| / 7\'7
| \ \   Xilinx Inc.
| / /
| \_\/.\   IBIS Models for VIRTEX-5
[IBIS ver]   3.2
[File name]   dlpc410.ibs
[File Rev]   1.8
[Date]   December 31, 2012
[Source]   Derived from spice models, rev0.20, dated 08/10/2005 using
   hspice 2005.03
[Notes]   Xilinx IBIS file for VIRTEX-5 I/O standards.
   All models are preliminary.
   The version of IBISCHK used is ibischk4.
   Ibis models were generated using S2IBIS3.
   To accurately model package parasitics, please include in
   your simulation a 50-65 ohm transmission line with 10-200ps of
   delay. For additional information, please see this Answer
   Record: http://support.xilinx.com/techdocs/11754.htm
   NOTE: This file is compliant with IBIS Version 3.2, but it
   may not implement all approved 3.2 features.
   NOTE:  Newer versions of the buffer models may be available.
   Check the web (http://www.xilinx.com/support/sw_ibis.htm) for
   the latest file revision.  However, please be aware that the
   web files are not compatible for use with IBISWriter, and
   must be manually annotated, should their use be preferred.
[Disclaimer] The data in this file is derived from SPICE simulations using
   modeling information extracted from the target process. While
   a great deal of care has been taken to provide information
   that is accurate, this model is considered preliminary as it
   has not been verified by actual silicon measurement. Treat the
   data in this model as preliminary until actual silicon
   verification is performed.
[Copyright]   Copyright 2006, Xilinx Inc., All rights reserved
|   Component VIRTEX-5
[Component]   VIRTEX-5
[Manufacturer]   Xilinx Inc.
[Package]
| For Package Type ff676
| variable   typ   min   max
R_pkg   253.6m   20.7m   604.1m
L_pkg   3.14nH   0.75nH   7.16nH
C_pkg   2.45pF   1.10pF   4.60pF
[Pin]  signal_name   model_name   R_pin   L_pin   C_pin
F7	APPS_CNTL_DPN   NC
E7 	APPS_CNTL_DPP   NC
AC13	ARSTZ   LVCMOS25_S_12_I
M14 	AVDD_0   NC
M13	AVSS_0   NC
E12 	BLKAD_0   LVCMOS25_S_12_I
D13	BLKAD_1   LVCMOS25_S_12_I
E13	BLKAD_2   LVCMOS25_S_12_I
F13	BLKAD_3   LVCMOS25_S_12_I
H13	BLKMD_0   LVCMOS25_S_12_I
H14	BLKMD_1   LVCMOS25_S_12_I
AD13	CLKIN_R   LVCMOS25_S_12_I
G19	COMP_DATA   LVCMOS25_S_12_I
N18	CS_B_0   NC
W11 	D_OUT_BUSY_0   NC
E1	DAD_A_ADDR0   LVCMOS25_F_12_O
E2	DAD_A_ADDR1   LVCMOS25_F_12_O
E3	DAD_A_ADDR2   LVCMOS25_F_12_O
F3 	DAD_A_ADDR3   LVCMOS25_F_12_O
C1	DAD_A_MODE0   LVCMOS25_F_12_O
D1	DAD_A_MODE1   LVCMOS25_F_12_O
AE3	DAD_A_SCPENZ   LVCMOS25_F_12_O
AB12	DAD_A_SEL0   LVCMOS25_F_12_O
AC12 	DAD_A_SEL1   LVCMOS25_F_12_O
AF3 	DAD_A_STROBE   LVCMOS25_F_12_O
E26	DAD_B_ADDR0   LVCMOS25_F_12_O
E25 	DAD_B_ADDR1   LVCMOS25_F_12_O
F25   DAD_B_ADDR2   LVCMOS25_F_12_O
F24	DAD_B_ADDR3   LVCMOS25_F_12_O
D26	DAD_B_MODE0   LVCMOS25_F_12_O
D25	DAD_B_MODE1   LVCMOS25_F_12_O
AB19	DAD_B_SCPENZ   LVCMOS25_F_12_O
R22	DAD_B_SEL0   LVCMOS25_F_12_O
R23	DAD_B_SEL1   LVCMOS25_F_12_O
AB20	DAD_B_STROBE   LVCMOS25_F_12_O
AF4	DAD_INIT   LVCMOS25_F_12_O
AF5	DAD_OEZ   LVCMOS25_F_12_O
L23	DDC_B11_VRN   NC
L22	DDC_B11_VRP   NC
C22	DDC_B11_VRP   NC
M5	DDC_B12_VRN   NC
M6	DDC_B12_VRP   NC
D23	DDC_B15_VRN   NC
A4	DDC_B16_VRN   NC
A5	DDC_B16_VRP   NC
B21	DDC_DCLK_A_DPN   LVDS_25
C21	DDC_DCLK_A_DPP   LVDS_25_I
A7	DDC_DCLK_B_DPN   LVDS_25
B7	DDC_DCLK_B_DPP  	LVDS_25_I
K20	DDC_DCLK_C_DPN   LVDS_25
K21	DDC_DCLK_C_DPP   LVDS_25_I
L5	DDC_DCLK_D_DPN   LVDS_25
K5	DDC_DCLK_D_DPP   LVDS_25_I
N1	DDC_DCLKOUT_A_DPN  	LVDS_25
M1 	DDC_DCLKOUT_A_DPP 	LVDS_25_O
Y5	DDC_DCLKOUT_B_DPN 	LVDS_25
Y6 	DDC_DCLKOUT_B_DPP 	LVDS_25_O
AA22	DDC_DCLKOUT_C_DPN 	LVDS_25
AB22	DDC_DCLKOUT_C_DPP  	LVDS_25_O
M26	DDC_DCLKOUT_D_DPN  	LVDS_25
M25 	DDC_DCLKOUT_D_DPP 	LVDS_25_O
A15	DDC_DIN_A0_DPN  	LVDS_25
A14	DDC_DIN_A0_DPP  	LVDS_25_I
B14 	DDC_DIN_A1_DPN  	LVDS_25
C14	DDC_DIN_A1_DPP  	LVDS_25_I
A22	DDC_DIN_A10_DPN 	LVDS_25
B22	DDC_DIN_A10_DPP   LVDS_25_I
A24	DDC_DIN_A11_DPN 	LVDS_25
A23	DDC_DIN_A11_DPP   LVDS_25_I
C23	DDC_DIN_A12_DPN 	LVDS_25
B24	DDC_DIN_A12_DPP   LVDS_25_I
C24	DDC_DIN_A13_DPN   LVDS_25
D24	DDC_DIN_A13_DPP 	LVDS_25_I
A25	DDC_DIN_A14_DPN 	LVDS_25
B25	DDC_DIN_A14_DPP 	LVDS_25_I
C26	DDC_DIN_A15_DPN 	LVDS_25
B26	DDC_DIN_A15_DPP 	LVDS_25_I
B16	DDC_DIN_A2_DPN  	LVDS_25
B15 	DDC_DIN_A2_DPP   LVDS_25_I
C16	DDC_DIN_A3_DPN  	LVDS_25
D16 	DDC_DIN_A3_DPP   LVDS_25_I
A17	DDC_DIN_A4_DPN  	LVDS_25
B17	DDC_DIN_A4_DPP  	LVDS_25_I
C17	DDC_DIN_A5_DPN  	LVDS_25
D18 	DDC_DIN_A5_DPP   LVDS_25_I
A19	DDC_DIN_A6_DPN  	LVDS_25
A18 	DDC_DIN_A6_DPP   LVDS_25_I
C18	DDC_DIN_A7_DPN   LVDS_25
B19	DDC_DIN_A7_DPP  	LVDS_25_I
D19	DDC_DIN_A8_DPN  	LVDS_25
C19 	DDC_DIN_A8_DPP   LVDS_25_I
B20	DDC_DIN_A9_DPN   LVDS_25
A20	DDC_DIN_A9_DPP   LVDS_25_I
A12	DDC_DIN_B0_DPN   LVDS_25
A13	DDC_DIN_B0_DPP   LVDS_25_I
B12	DDC_DIN_B1_DPN   LVDS_25
C13	DDC_DIN_B1_DPP   LVDS_25_I
B6	DDC_DIN_B10_DPN 	LVDS_25
B5	DDC_DIN_B10_DPP   LVDS_25_I
D4	DDC_DIN_B11_DPN 	LVDS_25
D3	DDC_DIN_B11_DPP  	LVDS_25_I
B4	DDC_DIN_B12_DPN 	LVDS_25
C4	DDC_DIN_B12_DPP 	LVDS_25_I
C3	DDC_DIN_B13_DPN   LVDS_25
C2	DDC_DIN_B13_DPP   LVDS_25_I
A3	DDC_DIN_B14_DPN  	LVDS_25
A2	DDC_DIN_B14_DPP   LVDS_25_I
B2	DDC_DIN_B15_DPN   LVDS_25
B1	DDC_DIN_B15_DPP   LVDS_25_I
D10	DDC_DIN_B2_DPN   LVDS_25
D11	DDC_DIN_B2_DPP   LVDS_25_I
C12	DDC_DIN_B3_DPN   LVDS_25
C11	DDC_DIN_B3_DPP   LVDS_25_I
A10	DDC_DIN_B4_DPN   LVDS_25
B11	DDC_DIN_B4_DPP   LVDS_25_I
D9	DDC_DIN_B5_DPN   LVDS_25
C9	DDC_DIN_B5_DPP   LVDS_25_I
B10	DDC_DIN_B6_DPN   LVDS_25
B9	DDC_DIN_B6_DPP   LVDS_25_I
A8	DDC_DIN_B7_DPN   LVDS_25
A9	DDC_DIN_B7_DPP   LVDS_25_I
D6	DDC_DIN_B8_DPN   LVDS_25
D5	DDC_DIN_B8_DPP   LVDS_25_I
C7	DDC_DIN_B9_DPN   LVDS_25
C6	DDC_DIN_B9_DPP   LVDS_25_I
E20	DDC_DIN_C0_DPN   LVDS_25
E21	DDC_DIN_C0_DPP   LVDS_25_I
F20	DDC_DIN_C1_DPN   LVDS_25
G20	DDC_DIN_C1_DPP  	LVDS_25_I
M19	DDC_DIN_C10_DPN  	LVDS_25
M20	DDC_DIN_C10_DPP  	LVDS_25_I
M21	DDC_DIN_C11_DPN   LVDS_25
M22	DDC_DIN_C11_DPP   LVDS_25_I
N19	DDC_DIN_C12_DPN   LVDS_25
P19	DDC_DIN_C12_DPP   LVDS_25_I
N21	DDC_DIN_C13_DPN   LVDS_25
N22	DDC_DIN_C13_DPP  	LVDS_25_I
P20	DDC_DIN_C14_DPN   LVDS_25
P21	DDC_DIN_C14_DPP  	LVDS_25_I
N23	DDC_DIN_C15_DPN   LVDS_25
P23	DDC_DIN_C15_DPP   LVDS_25_I
H19	DDC_DIN_C2_DPN  	LVDS_25
J19	DDC_DIN_C2_DPP   LVDS_25_I
E23	DDC_DIN_C3_DPN   LVDS_25
E22	DDC_DIN_C3_DPP   LVDS_25_I
F23	DDC_DIN_C4_DPN   LVDS_25
F22	DDC_DIN_C4_DPP   LVDS_25_I
G22	DDC_DIN_C5_DPN   LVDS_25
G21	DDC_DIN_C5_DPP   LVDS_25_I
J20	DDC_DIN_C6_DPN   LVDS_25
J21	DDC_DIN_C6_DPP   LVDS_25_I
H22	DDC_DIN_C7_DPN   LVDS_25
H21	DDC_DIN_C7_DPP   LVDS_25_I
J23	DDC_DIN_C8_DPN   LVDS_25
H23	DDC_DIN_C8_DPP   LVDS_25_I
K22	DDC_DIN_C9_DPN   LVDS_25
K23	DDC_DIN_C9_DPP   LVDS_25_I
T3	DDC_DIN_D0_DPN  	LVDS_25
R3	DDC_DIN_D0_DPP   LVDS_25_I
R5	DDC_DIN_D1_DPN   LVDS_25
R6	DDC_DIN_D1_DPP   LVDS_25_I
H7	DDC_DIN_D10_DPN   LVDS_25
J6	DDC_DIN_D10_DPP 	LVDS_25_I
G4	DDC_DIN_D11_DPN   LVDS_25
H4	DDC_DIN_D11_DPP   LVDS_25_I
G5	DDC_DIN_D12_DPN   LVDS_25
H6	DDC_DIN_D12_DPP 	LVDS_25_I
G7	DDC_DIN_D13_DPN   LVDS_25
G6	DDC_DIN_D13_DPP 	LVDS_25_I
F4	DDC_DIN_D14_DPN  	LVDS_25
F5	DDC_DIN_D14_DPP  	LVDS_25_I
E5	DDC_DIN_D15_DPN   LVDS_25
E6	DDC_DIN_D15_DPP   LVDS_25_I
R7	DDC_DIN_D2_DPN  	LVDS_25
P6	DDC_DIN_D2_DPP   LVDS_25_I
N3	DDC_DIN_D3_DPN   LVDS_25
P3	DDC_DIN_D3_DPP  	LVDS_25_I
P4	DDC_DIN_D4_DPN   LVDS_25
P5	DDC_DIN_D4_DPP   LVDS_25_I
N6	DDC_DIN_D5_DPN   LVDS_25
N7	DDC_DIN_D5_DPP  	LVDS_25_I
N4	DDC_DIN_D6_DPN   LVDS_25
M4	DDC_DIN_D6_DPP  	LVDS_25_I
M7	DDC_DIN_D7_DPN   LVDS_25
L7	DDC_DIN_D7_DPP   LVDS_25_I
K7	DDC_DIN_D8_DPN   LVDS_25
K6	DDC_DIN_D8_DPP   LVDS_25_I
J4	DDC_DIN_D9_DPN   LVDS_25
J5	DDC_DIN_D9_DPP   LVDS_25_I
AE2	DDC_DOUT_A0_DPN 	LVDS_25
AF2	DDC_DOUT_A0_DPP 	LVDS_25_O
AD1	DDC_DOUT_A1_DPN  	LVDS_25
AE1	DDC_DOUT_A1_DPP 	LVDS_25_O
K1	DDC_DOUT_A10_DPN 	LVDS_25
L2	DDC_DOUT_A10_DPP 	LVDS_25_O
K2	DDC_DOUT_A11_DPN 	LVDS_25
K3	DDC_DOUT_A11_DPP 	LVDS_25_O
J3	DDC_DOUT_A12_DPN 	LVDS_25
H3	DDC_DOUT_A12_DPP	LVDS_25_O
H2	DDC_DOUT_A13_DPN	LVDS_25
J1	DDC_DOUT_A13_DPP	LVDS_25_O
H1	DDC_DOUT_A14_DPN	LVDS_25
G1	DDC_DOUT_A14_DPP 	LVDS_25_O
G2	DDC_DOUT_A15_DPN 	LVDS_25
F2	DDC_DOUT_A15_DPP 	LVDS_25_O
AC1	DDC_DOUT_A2_DPN   LVDS_25
AC2	DDC_DOUT_A2_DPP   LVDS_25_O
AB1	DDC_DOUT_A3_DPN   LVDS_25
AB2	DDC_DOUT_A3_DPP   LVDS_25_O
Y2	DDC_DOUT_A4_DPN   LVDS_25
AA2	DDC_DOUT_A4_DPP   LVDS_25_O
W1	DDC_DOUT_A5_DPN   LVDS_25
Y1	DDC_DOUT_A5_DPP   LVDS_25_O
V1	DDC_DOUT_A6_DPN 	LVDS_25
V2	DDC_DOUT_A6_DPP   LVDS_25_O
U1	DDC_DOUT_A7_DPN   LVDS_25
U2	DDC_DOUT_A7_DPP   LVDS_25_O
R2	DDC_DOUT_A8_DPN   LVDS_25
T2	DDC_DOUT_A8_DPP   LVDS_25_O
N2	DDC_DOUT_A9_DPN 	LVDS_25
M2	DDC_DOUT_A9_DPP   LVDS_25_O
AE5	DDC_DOUT_B0_DPN   LVDS_25
AE6	DDC_DOUT_B0_DPP   LVDS_25_O
AD3	DDC_DOUT_B1_DPN   LVDS_25
AD4	DDC_DOUT_B1_DPP   LVDS_25_O
W6	DDC_DOUT_B10_DPN  	LVDS_25
W5	DDC_DOUT_B10_DPP 	LVDS_25_O
V7	DDC_DOUT_B11_DPN 	LVDS_25
V6	DDC_DOUT_B11_DPP	LVDS_25_O
U4	DDC_DOUT_B12_DPN 	LVDS_25
V3	DDC_DOUT_B12_DPP	LVDS_25_O
T4	DDC_DOUT_B13_DPN 	LVDS_25
T5	DDC_DOUT_B13_DPP 	LVDS_25_O
U6	DDC_DOUT_B14_DPN 	LVDS_25
U5	DDC_DOUT_B14_DPP	LVDS_25_O
U7	DDC_DOUT_B15_DPN	LVDS_25
T7	DDC_DOUT_B15_DPP 	LVDS_25_O
AD5	DDC_DOUT_B2_DPN 	LVDS_25
AD6   DDC_DOUT_B2_DPP   LVDS_25_O
AC3	DDC_DOUT_B3_DPN 	LVDS_25
AC4	DDC_DOUT_B3_DPP 	LVDS_25_O
AB5	DDC_DOUT_B4_DPN 	LVDS_25
AB6	DDC_DOUT_B4_DPP   LVDS_25_O
AB7	DDC_DOUT_B5_DPN   LVDS_25
AC6	DDC_DOUT_B5_DPP   LVDS_25_O
AA5	DDC_DOUT_B6_DPN   LVDS_25
AA4	DDC_DOUT_B6_DPP   LVDS_25_O
AA7	DDC_DOUT_B7_DPN   LVDS_25
Y7	DDC_DOUT_B7_DPP   LVDS_25_O
Y3	DDC_DOUT_B8_DPN   LVDS_25
W3	DDC_DOUT_B8_DPP   LVDS_25_O
W4	DDC_DOUT_B9_DPN 	LVDS_25
V4	DDC_DOUT_B9_DPP 	LVDS_25_O
T22	DDC_DOUT_C0_DPN   LVDS_25
T23	DDC_DOUT_C0_DPP   LVDS_25_O
R20	DDC_DOUT_C1_DPN   LVDS_25
R21	DDC_DOUT_C1_DPP   LVDS_25_O
Y20	DDC_DOUT_C10_DPN	LVDS_25
Y21	DDC_DOUT_C10_DPP	LVDS_25_O
AA24	DDC_DOUT_C11_DPN	LVDS_25
AA23	DDC_DOUT_C11_DPP	LVDS_25_O
AA19	DDC_DOUT_C12_DPN	LVDS_25
AA20	DDC_DOUT_C12_DPP	LVDS_25_O
AC24	DDC_DOUT_C13_DPN	LVDS_25
AB24	DDC_DOUT_C13_DPP  	LVDS_25_O
AC19	DDC_DOUT_C14_DPN	LVDS_25
AD19	DDC_DOUT_C14_DPP	LVDS_25_O
AC22	DDC_DOUT_C15_DPN	LVDS_25
AC23	DDC_DOUT_C15_DPP	LVDS_25_O
T19	DDC_DOUT_C2_DPN   LVDS_25
T20	DDC_DOUT_C2_DPP   LVDS_25_O
U21	DDC_DOUT_C3_DPN 	LVDS_25
U22	DDC_DOUT_C3_DPP   LVDS_25_O
U20	DDC_DOUT_C4_DPN   LVDS_25
U19	DDC_DOUT_C4_DPP   LVDS_25_O
V23	DDC_DOUT_C5_DPN   LVDS_25
V24	DDC_DOUT_C5_DPP 	LVDS_25_O
V22	DDC_DOUT_C6_DPN 	LVDS_25
V21	DDC_DOUT_C6_DPP   LVDS_25_O
W19	DDC_DOUT_C7_DPN   LVDS_25
V19	DDC_DOUT_C7_DPP 	LVDS_25_O
W23	DDC_DOUT_C8_DPN   LVDS_25
W24	DDC_DOUT_C8_DPP   LVDS_25_O
Y22	DDC_DOUT_C9_DPN 	LVDS_25
Y23	DDC_DOUT_C9_DPP   LVDS_25_O
AB26	DDC_DOUT_D0_DPN   LVDS_25
AC26	DDC_DOUT_D0_DPP   LVDS_25_O
AA25	DDC_DOUT_D1_DPN 	LVDS_25
AB25	DDC_DOUT_D1_DPP   LVDS_25_O
L25	DDC_DOUT_D10_DPN 	LVDS_25
L24	DDC_DOUT_D10_DPP	LVDS_25_O
K26	DDC_DOUT_D11_DPN 	LVDS_25
K25	DDC_DOUT_D11_DPP	LVDS_25_O
J26	DDC_DOUT_D12_DPN 	LVDS_25
J25	DDC_DOUT_D12_DPP  	LVDS_25_O
J24	DDC_DOUT_D13_DPN   LVDS_25
H24	DDC_DOUT_D13_DPP	LVDS_25_O
H26	DDC_DOUT_D14_DPN	LVDS_25
G26	DDC_DOUT_D14_DPP	LVDS_25_O
G25	DDC_DOUT_D15_DPN	LVDS_25
G24	DDC_DOUT_D15_DPP 	LVDS_25_O
Y26	DDC_DOUT_D2_DPN   LVDS_25
Y25	DDC_DOUT_D2_DPP 	LVDS_25_O
W26	DDC_DOUT_D3_DPN   LVDS_25
W25	DDC_DOUT_D3_DPP   LVDS_25_O
U26	DDC_DOUT_D4_DPN   LVDS_25
V26	DDC_DOUT_D4_DPP   LVDS_25_O
U25	DDC_DOUT_D5_DPN  	LVDS_25
U24	DDC_DOUT_D5_DPP   LVDS_25_O
T25	DDC_DOUT_D6_DPN 	LVDS_25
T24	DDC_DOUT_D6_DPP  	LVDS_25_O
R26	DDC_DOUT_D7_DPN   LVDS_25
R25	DDC_DOUT_D7_DPP  	LVDS_25_O
P24	DDC_DOUT_D8_DPN  	LVDS_25
P25	DDC_DOUT_D8_DPP   LVDS_25_O
N24	DDC_DOUT_D9_DPN   LVDS_25
M24	DDC_DOUT_D9_DPP   LVDS_25_O
W18	DDC_M0   NC
Y17	DDC_M1   NC
V18	DDC_M2   NC
R1	DDC_SCTRL_AN   LVDS_25
P1	DDC_SCTRL_AP   LVDS_25_O
AA3	DDC_SCTRL_BN   LVDS_25
AB4	DDC_SCTRL_BP   LVDS_25_O
W20	DDC_SCTRL_CN   LVDS_25
W21	DDC_SCTRL_CP   LVDS_25_O
N26	DDC_SCTRL_DN   LVDS_25
P26	DDC_SCTRL_DP   LVDS_25_O
AB21	DDC_SPARE_0   LVCMOS25_F_12_O
AC21	DDC_SPARE_1   LVCMOS25_F_12_O
F18	DDC_VERSION_0   LVCMOS25_F_12_O
G17	DDC_VERSION_1   LVCMOS25_F_12_O
H18	DDC_VERSION_2   LVCMOS25_F_12_O
AD14	DMD_A_RESET   LVCMOS25_F_12_O
AB14	DMD_A_SCPENZ   LVCMOS25_F_12_O
AA12	DMD_B_RESET   LVCMOS25_S_12
AC14	DMD_B_SCPENZ   NC
AA17	DMD_TYPE_0   LVCMOS25_F_12_O
AC16	DMD_TYPE_1   LVCMOS25_F_12_O
AB17	DMD_TYPE_2   LVCMOS25_F_12_O
AD15	DMD_TYPE_3   LVCMOS25_F_12_O
K10	DONE_DDC   NC
D20	DVALID_A_DPN   LVDS_25
D21	DVALID_A_DPP   LVDS_25_I
C8	DVALID_B_DPN   LVDS_25
D8	DVALID_B_DPP   LVDS_25_I
L19	DVALID_C_DPN   LVDS_25
L20	DVALID_C_DPP   LVDS_25_I
L3	DVALID_D_DPN   LVDS_25
L4	DVALID_D_DPP   LVDS_25_I
R13	DXN_0   NC
R14	DXP_0   NC
Y18	ECP2_FINISHED   LVCMOS25_F_12_O
AD11	ECP2_M_TP0   NC
AD10	ECP2_M_TP1   NC
AB10 	ECP2_M_TP10   LVCMOS25_F_12_O
AA10 	ECP2_M_TP11   LVCMOS25_F_12_O
Y10	ECP2_M_TP12   LVCMOS25_F_12_O
AC11 	ECP2_M_TP13   LVCMOS25_F_12_O
Y12	ECP2_M_TP14   LVCMOS25_F_12_O
Y11	ECP2_M_TP15   LVCMOS25_F_12_O
AB11	ECP2_M_TP16   LVCMOS25_F_12_O
H8 	ECP2_M_TP17   LVCMOS25_F_12_O
H9	ECP2_M_TP18   LVCMOS25_F_12_O
F12	ECP2_M_TP19   LVCMOS25_F_12_O
AD8	ECP2_M_TP2   NC
G11	ECP2_M_TP20   LVCMOS25_F_12_O
G12	ECP2_M_TP21   LVCMOS25_F_12_O
E11  	ECP2_M_TP22   LVCMOS25_F_12_O
E10	ECP2_M_TP23   LVCMOS25_F_12_O
E8 	ECP2_M_TP24   LVCMOS25_F_12_O
F10	ECP2_M_TP25   LVCMOS25_F_12_O
F9 	ECP2_M_TP26   LVCMOS25_F_12_O
F8	ECP2_M_TP27   LVCMOS25_F_12_O
G10	ECP2_M_TP28   LVCMOS25_F_12_O
G9	ECP2_M_TP29   LVCMOS25_F_12_O
AC8	ECP2_M_TP3   LVCMOS25_F_12_O
H11	ECP2_M_TP30   LVCMOS25_F_12_O
H12 	ECP2_M_TP31   LVCMOS25_F_12_O
AC7	ECP2_M_TP4   LVCMOS25_F_12_O
AC9	ECP2_M_TP5   LVCMOS25_F_12_O
AB9	ECP2_M_TP6   LVCMOS25_F_12_O
AA8	ECP2_M_TP7   LVCMOS25_F_12_O
AA9	ECP2_M_TP8   LVCMOS25_F_12_O
Y8  	ECP2_M_TP9   LVCMOS25_F_12_O
A1   GND   GND
A11   GND   GND
A16   GND   GND
A21   GND   GND
A26   GND   GND
A6   GND   GND
AA1   GND   GND
AA11   GND   GND
AA21   GND   GND
AA26   GND   GND
AB18   GND   GND
AB8   GND   GND
AC15   GND   GND
AC25   GND   GND
AC5   GND   GND
AD12   GND   GND
AD2   GND   GND
AD22   GND   GND
AE14   GND   GND
AE19   GND   GND
AE4   GND   GND
AE9   GND   GND
AF1   GND   GND
AF11   GND   GND
AF16   GND   GND
AF21   GND   GND
AF26   GND   GND
AF6   GND   GND
B13   GND   GND
B18   GND   GND
B3   GND   GND
B8   GND   GND
C15   GND   GND
C25   GND   GND
C5   GND   GND
D12   GND   GND
D2   GND   GND
D22   GND   GND
E19   GND   GND
E9   GND   GND
F1   GND   GND
F16   GND   GND
F26   GND   GND
F6   GND   GND
G13   GND   GND
G18   GND   GND
G23   GND   GND
G3   GND   GND
H10   GND   GND
H20   GND   GND
J13   GND   GND
J15   GND   GND
J17   GND   GND
J7   GND   GND
J9   GND   GND
K12   GND   GND
K14   GND   GND
K16   GND   GND
K19   GND   GND
K24   GND   GND
K4   GND   GND
K8   GND   GND
L1   GND   GND
L11   GND   GND
L13   GND   GND
L15   GND   GND
L17   GND   GND
L21   GND   GND
L26   GND   GND
L9   GND   GND
M10   GND   GND
M12   GND   GND
M16   GND   GND
M18   GND   GND
M3   GND   GND
M8   GND   GND
N11   GND   GND
N15   GND   GND
N17   GND   GND
N25   GND   GND
N5   GND   GND
N9   GND   GND
P10   GND   GND
P12   GND   GND
P16   GND   GND
P2   GND   GND
P22   GND   GND
P7   GND   GND
P8   GND   GND
R11   GND   GND
R15   GND   GND
R17   GND   GND
R19   GND   GND
R9   GND   GND
T1   GND   GND
T10   GND   GND
T12   GND   GND
T14   GND   GND
T16   GND   GND
T26   GND   GND
T6   GND   GND
T8   GND   GND
U13   GND   GND
U15   GND   GND
U17   GND   GND
U18   GND   GND
U23   GND   GND
U3   GND   GND
U9   GND   GND
V10   GND   GND
V14   GND   GND
V16   GND   GND
V20   GND   GND
V8   GND   GND
W13   GND   GND
W15   GND   GND
W17   GND   GND
W7   GND   GND
W9   GND   GND
Y14   GND   GND
Y16   GND   GND
Y19   GND   GND
Y24   GND   GND
Y4   GND   GND
L18  	HSWAPEN   NC
AA18   INIT_ACTIVE   LVCMOS25_F_12_O
J11	INTB_DDC   NC
F19	NS_FLIP   LVCMOS25_S_12_I
J18	PROGB_DDC   NC
J10   PROM_CCK_DDC   LVCMOS25_S_12
K11 	PROM_D0_DDC   NC
AC17   PWR_FLOAT   LVCMOS25_S_12_I
P18	RDWR_B   NC
D14   ROWAD_0   LVCMOS25_S_12_I
D15   ROWAD_1   LVCMOS25_S_12_I
G16 	ROWAD_10   LVCMOS25_S_12_I
E15  	ROWAD_2   LVCMOS25_S_12_I
F14   ROWAD_3   LVCMOS25_S_12_I
G14   ROWAD_4   LVCMOS25_S_12_I
E16   ROWAD_5   LVCMOS25_S_12_I
F15   ROWAD_6   LVCMOS25_S_12_I
G15	ROWAD_7   LVCMOS25_S_12_I
E17	ROWAD_8   LVCMOS25_S_12_I
F17   ROWAD_9   LVCMOS25_S_12_I
H17   ROWMD_0   LVCMOS25_S_12_I
H16   ROWMD_1   LVCMOS25_S_12_I
AB16   RST_ACTIVE   LVCMOS25_F_12_O
E18 	RST2BLKZ   LVCMOS25_S_12_I
R18	RSVD_0   NC
T18 	RSVD_0   NC
AB15   SCPCLK   LVCMOS25_F_12_O
AA15   SCPDI   LVCMOS25_S_12_I
AA14   SCPDO   LVCMOS25_F_12_O
Y13   STEPVCC   LVCMOS25_S_12_I
U11   TCK_JTAG   NC
W10   TDO_DDC   NC
V11 	TDO_XCF16DDC   NC
V12	TMS_JTAG   NC
K18 	VBATT_0   NC
J8   VCCAUX   POWER
K17   VCCAUX   POWER
L8   VCCAUX   POWER
M17   VCCAUX   POWER
N8   VCCAUX   POWER
P17   VCCAUX   POWER
R8   VCCAUX   POWER
T17   VCCAUX   POWER
U8   VCCAUX   POWER
V17   VCCAUX   POWER
W16   VCCAUX   POWER
W8   VCCAUX   POWER
H15   VCCINT   POWER
J12   VCCINT   POWER
J14   VCCINT   POWER
J16   VCCINT   POWER
K13   VCCINT   POWER
K15   VCCINT   POWER
K9   VCCINT   POWER
L10   VCCINT   POWER
L12   VCCINT   POWER
L14   VCCINT   POWER
L16   VCCINT   POWER
M11   VCCINT   POWER
M15   VCCINT   POWER
M9   VCCINT   POWER
N10   VCCINT   POWER
N12   VCCINT   POWER
N16   VCCINT   POWER
P11   VCCINT   POWER
P15   VCCINT   POWER
P9   VCCINT   POWER
R10   VCCINT   POWER
R12   VCCINT   POWER
R16   VCCINT   POWER
T11   VCCINT   POWER
T13   VCCINT   POWER
T15   VCCINT   POWER
T9   VCCINT   POWER
U10   VCCINT   POWER
U12   VCCINT   POWER
U14   VCCINT   POWER
U16   VCCINT   POWER
V13   VCCINT   POWER
V15   VCCINT   POWER
V9   VCCINT   POWER
W14   VCCINT   POWER
Y15   VCCINT   POWER
W12   VCCO_0   POWER
Y9   VCCO_0   POWER
C10   VCCO_1   POWER
F11   VCCO_1   POWER
F21   VCCO_11   POWER
H25   VCCO_11   POWER
J22   VCCO_11   POWER
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[Diff Pin]   inv_pin   vdiff   tdelay_typ   tdelay_min   tdelay_max
[Package Model] ff676_xc5vlx30
[Define Package Model]   ff676_xc5vlx30
[Manufacturer]   Xilinx Inc.
[OEM]   Xilinx_K1
[Description]   676 ball organic flipchip
[Number Of Pins]   444
[Pin Numbers]
P20   | 1   P20   D1.245   IO_L19N_SM9N_11
AC17   | 2   AC17  D1.164   IO_L2P_GC_D11_4
F18   | 3   F18   D1.145   IO_L9P_GC_3
B12   | 4   B12   D1.534   IO_L2N_16
T19   | 5   T19   D1.603   IO_L2N_17
H1   | 6   H1   D1.399   IO_L2N_14
B16   | 7   B16   D1.468   IO_L2N_15
G7   | 8   G7   D1.264   IO_L2N_12
E23   | 9   E23   D1.198   IO_L2N_11
K25   | 10   K25   D1.342   IO_L7P_SM2P_13
U6   | 11   U6   D1.671   IO_L3N_18
U21   | 12   U21   D1.605   IO_L3N_17
A12   | 13   A12   D1.536   IO_L3N_16
C16   | 14   C16   D1.470   IO_L3N_15
G2   | 15   G2   D1.401   IO_L3N_14
F4   | 16   F4   D1.266   IO_L3N_12
F23   | 17   F23   D1.200   IO_L3N_11
F10   | 18   F10   D1.140   IO_L6N_GC_3
J18   | 19   J18   D1.26   PROGRAM_B_0
E8   | 20   E8   D1.144   IO_L8N_GC_3
AC4   | 21   AC4   D1.702   IO_L12P_VRN_18
R25   | 22   R25   D1.365   IO_L12P_VRN_13
M5   | 23   M5   D1.297   IO_L12P_VRN_12
L23   | 24   L23   D1.230   IO_L12P_VRN_11
V21   | 25   V21   D1.635   IO_L12P_VRN_17
A4   | 26   A4   D1.567   IO_L12P_VRN_16
D23   | 27   D23   D1.500   IO_L12P_VRN_15
U2   | 28   U2   D1.432   IO_L12P_VRN_14
K22   | 29   K22   D1.227   IO_L10N_CC_SM15N_11
U7   | 30   U7   D1.669   IO_L2N_18
W12   | 31   W12   D1.35   VCCO_0
C10   | 32   C10   C3.1   VCCO_1
AA16   | 33   AA16  C15.2   VCCO_2
D17   | 34   D17   C4.1   VCCO_3
AB13   | 35   AB13  C16.2   VCCO_4
W11   | 36   W11   D1.59   D_OUT_BUSY_0
M21   | 37   M21   D1.233   IO_L13N_11
T25   | 38   T25   D1.368   IO_L13N_13
N6   | 39   N6   D1.300   IO_L13N_12
A22   | 40   A22   D1.503   IO_L13N_15
V1   | 41   V1   D1.435   IO_L13N_14
W20   | 42   W20   D1.638   IO_L13N_17
B6   | 43   B6   D1.570   IO_L13N_16
L25   | 44   L25   D1.341   IO_L6N_SM3N_13
F19   | 45   F19   D1.142   IO_L7N_GC_3
Y18   | 46   Y18   D1.97   IO_L1N_CC_A24_2
W4   | 47   W4   D1.673   IO_L4N_VREF_18
W24   | 48   W24   D1.606   IO_L4P_17
J26   | 49   J26   D1.337   IO_L4N_VREF_13
H7   | 50   H7   D1.268   IO_L4N_VREF_12
G22   | 51   G22   D1.202   IO_L4N_VREF_11
W23   | 52   W23   D1.607   IO_L4N_VREF_17
D9   | 53   D9   D1.538   IO_L4N_VREF_16
C17   | 54   C17   D1.472   IO_L4N_VREF_15
K2   | 55   K2   D1.403   IO_L4N_VREF_14
H23   | 56   H23   D1.207   IO_L7P_11
J25   | 57   J25   D1.336   IO_L4P_13
U11   | 58   U11   D1.51   TCK_0
J10   | 59   J10   D1.30   CCLK_0
N14   | 60   N14   D1.16   VP_0
AA19   | 61   AA19  D1.650   IO_L19N_17
B2   | 62   B2   D1.582   IO_L19N_16
D25   | 63   D25   D1.515   IO_L19N_15
AE2   | 64   AE2   D1.447   IO_L19N_14
AB26   | 65   AB26  D1.380   IO_L19N_13
R7   | 66   R7   D1.312   IO_L19N_12
G19   | 67   G19   D1.77   IO_L8P_CC_A3_D19_1
AE5   | 68   AE5   D1.717   IO_L19N_18
R4   | 69   R4   C20.1   VCCO_14
G24   | 70   G24   D1.334   IO_L3P_SM5P_13
K11   | 71   K11   D1.28   D_IN_0
B19   | 72   B19   D1.477   IO_L7P_15
AA7   | 73   AA7   D1.699   IO_L10N_CC_18
AC18   | 74   AC18  D1.161   IO_L0N_GC_D14_4
P13   | 75   P13   D1.17   VN_0
AA8   | 76   AA8   D1.99   IO_L2N_A22_2
L5   | 77   L5   D1.294   IO_L10N_CC_12
N26   | 78   N26   D1.362   IO_L10N_CC_13
D6   | 79   D6   D1.564   IO_L10N_CC_16
AA22   | 80   AA22  D1.632   IO_L10N_CC_17
R1   | 81   R1   D1.429   IO_L10N_CC_14
D20   | 82   D20   D1.497   IO_L10N_CC_15
AC14   | 83   AC14  D1.173   IO_L6N_GC_4
F5   | 84   F5   D1.265   IO_L3P_12
D16   | 85   D16   D1.469   IO_L3P_15
P23   | 86   P23   D1.238   IO_L16P_SM12P_11
J5   | 87   J5   D1.273   IO_L7P_12
R18   | 88   R18   D1.38   VFS_0
C24   | 89   C24   D1.509   IO_L16N_15
F12   | 90   F12   D1.132   IO_L2N_GC_VRP_3
H5   | 91   H5   C22.1   VCCO_12
M23   | 92   M23   C9.2   VCCO_13
F21   | 93   F21   C8.2   VCCO_11
D7   | 94   D7   C1.1   VCCO_16
T21   | 95   T21   C11.2   VCCO_17
H14   | 96   H14   D1.63   IO_L1P_A17_1
B23   | 97   B23   C6.1   VCCO_15
AA6   | 98   AA6   C18.2   VCCO_18
K23   | 99   K23   D1.226   IO_L10P_CC_SM15P_11
AD18   | 100   AD18  D1.160   IO_L0P_GC_D15_4
AD4   | 101   AD4   D1.704   IO_L13P_18
K26   | 102   K26   D1.343   IO_L7N_SM2N_13
U24   | 103   U24   D1.371   IO_L15P_13
M4   | 104   M4   D1.303   IO_L15P_12
B24   | 105   B24   D1.506   IO_L15P_15
AA2   | 106   AA2   D1.438   IO_L15P_14
V19   | 107   V19   D1.641   IO_L15P_17
C4   | 108   C4   D1.573   IO_L15P_16
AC6   | 109   AC6   D1.708   IO_L15P_18
C7   | 110   C7   D1.566   IO_L11N_CC_16
V18   | 111   V18   D1.55   M2_0
G25   | 112   G25   D1.335   IO_L3N_SM5N_13
G15   | 113   G15   D1.66   IO_L2N_A14_D30_1
J20   | 114   J20   D1.210   IO_L8N_CC_11
K7   | 115   K7   D1.276   IO_L8N_CC_12
N1   | 116   N1   D1.411   IO_L8N_CC_14
B20   | 117   B20   D1.480   IO_L8N_CC_15
C8   | 118   C8   D1.546   IO_L8N_CC_16
AB9   | 119   AB9   D1.163   IO_L1N_GC_D12_4
Y5   | 120   Y5   D1.681   IO_L8N_CC_18
AB12   | 121   AB12  D1.174   IO_L7P_GC_VRN_4
AC12   | 122   AC12  D1.177   IO_L8N_CC_GC_4
AF5   | 123   AF5   D1.714   IO_L18P_18
R6   | 124   R6   D1.309   IO_L18P_12
AB25   | 125   AB25  D1.377   IO_L18P_13
AE1   | 126   AE1   D1.444   IO_L18P_14
B26   | 127   B26   D1.512   IO_L18P_15
D1   | 128   D1   D1.579   IO_L18P_16
AB20   | 129   AB20  D1.647   IO_L18P_17
L19   | 130   L19   D1.229   IO_L11N_CC_SM14N_11
H8   | 131   H8   D1.80   IO_L9N_CC_A0_D16_1
AC9   | 132   AC9   D1.167   IO_L3N_GC_D8_4
K10   | 133   K10   D1.29   DONE_0
G26   | 134   G26   D1.332   IO_L2P_SM6P_13
J8   | 135   J8   C10.2   VCCAUX
U25   | 136   U25   D1.372   IO_L15N_13
AA14   | 137   AA14  D1.113   IO_L9N_D0_FS0_2
Y17   | 138   Y17   D1.56   M1_0
W19   | 139   W19   D1.642   IO_L15N_17
B4   | 140   B4   D1.574   IO_L15N_16
C23   | 141   C23   D1.507   IO_L15N_15
Y2   | 142   Y2   D1.439   IO_L15N_14
AB7   | 143   AB7   D1.709   IO_L15N_18
AB6   | 144   AB6   D1.706   IO_L14P_18
Y1   | 145   Y1   D1.436   IO_L14P_14
A23   | 146   A23   D1.504   IO_L14P_15
D3   | 147   D3   D1.571   IO_L14P_16
U19   | 148   U19   D1.639   IO_L14P_17
P19   | 149   P19   D1.234   IO_L14P_11
P3   | 150   P3   D1.301   IO_L14P_12
V26   | 151   V26   D1.369   IO_L14P_13
AD19   | 152   AD19  D1.645   IO_L17P_17
A2   | 153   A2   D1.577   IO_L17P_16
B25   | 154   B25   D1.510   IO_L17P_15
AC2   | 155   AC2   D1.442   IO_L17P_14
Y25   | 156   Y25   D1.375   IO_L17P_13
R3   | 157   R3   D1.307   IO_L17P_12
N22   | 158   N22   D1.240   IO_L17P_SM11P_11
AD6   | 159   AD6   D1.712   IO_L17P_18
AC20   | 160   AC20  B1.AB23   VCCO_21
D15   | 161   D15   D1.133   IO_L3P_GC_3
J11   | 162   J11   D1.31   INIT_B_0
J24   | 163   J24   D1.339   IO_L5N_SM4N_13
M13   | 164   M13   D1.12   AVSS_0
T18   | 165   T18   D1.44   R_FUSE_0
G9   | 166   G9   D1.76   IO_L7N_A4_D20_1
V7   | 167   V7   D1.677   IO_L6N_18
G4   | 168   G4   D1.272   IO_L6N_12
H19   | 169   H19   D1.206   IO_L6N_11
A10   | 170   A10   D1.542   IO_L6N_16
AA24   | 171   AA24  D1.611   IO_L6N_17
K1   | 172   K1   D1.407   IO_L6N_14
A19   | 173   A19   D1.476   IO_L6N_15
F17   | 174   F17   D1.146   IO_L9N_GC_3
G14   | 175   G14   D1.61   IO_L0P_A19_1
AA10   | 176   AA10  D1.102   IO_L4P_FCS_B_2
AD3   | 177   AD3   D1.705   IO_L13N_18
W6   | 178   W6   D1.679   IO_L7N_18
J4   | 179   J4   D1.274   IO_L7N_12
J23   | 180   J23   D1.208   IO_L7N_11
Y22   | 181   Y22   D1.613   IO_L7N_17
A8   | 182   A8   D1.544   IO_L7N_16
C18   | 183   C18   D1.478   IO_L7N_15
H2   | 184   H2   D1.409   IO_L7N_14
F25   | 185   F25   D1.329   IO_L0N_SM8N_13
AC22   | 186   AC22  D1.615   IO_L8N_CC_17
Y11   | 187   Y11   D1.95   IO_L0N_CC_RS0_2
AC8   | 188   AC8   D1.166   IO_L3P_GC_D9_4
V12   | 189   V12   D1.57   TMS_0
M25   | 190   M25   D1.344   IO_L8P_CC_SM1P_13
A24   | 191   A24   D1.505   IO_L14N_VREF_15
W1   | 192   W1   D1.437   IO_L14N_VREF_14
U20   | 193   U20   D1.640   IO_L14N_VREF_17
D4   | 194   D4   D1.572   IO_L14N_VREF_16
N19   | 195   N19   D1.235   IO_L14N_VREF_11
U26   | 196   U26   D1.370   IO_L14N_VREF_13
N3   | 197   N3   D1.302   IO_L14N_VREF_12
T24   | 198   T24   D1.367   IO_L13P_13
N7   | 199   N7   D1.299   IO_L13P_12
M22   | 200   M22   D1.232   IO_L13P_11
W21   | 201   W21   D1.637   IO_L13P_17
AB5   | 202   AB5   D1.707   IO_L14N_VREF_18
B22   | 203   B22   D1.502   IO_L13P_15
V2   | 204   V2   D1.434   IO_L13P_14
H18   | 205   H18   D1.78   IO_L8N_CC_A2_D18_1
F24   | 206   F24   D1.328   IO_L0P_SM8P_13
P14   | 207   P14   D1.18   VREFP_0
R23   | 208   R23   D1.243   IO_L18N_SM10N_11
H17   | 209   H17   D1.73   IO_L6P_A7_D23_1
W18   | 210   W18   D1.54   M0_0
AE6   | 211   AE6   D1.716   IO_L19P_18
G11   | 212   G11   D1.72   IO_L5N_A8_D24_1
H24   | 213   H24   D1.338   IO_L5P_SM4P_13
E13   | 214   E13   D1.128   IO_L0N_CC_GC_3
Y10   | 215   Y10   D1.94   IO_L0P_CC_RS1_2
B1   | 216   B1   D1.581   IO_L19P_16
R13   | 217   R13   D1.6   DXN_0
P21   | 218   P21   D1.244   IO_L19P_SM9P_11
B21   | 219   B21   D1.499   IO_L11N_CC_15
K18   | 220   K18   D1.25   VBATT_0
R2   | 221   R2   D1.431   IO_L11N_CC_14
AA12   | 222   AA12  D1.110   IO_L8P_D3_2
A14   | 223   A14   D1.465   IO_L1P_15
F14   | 224   F14   D1.127   IO_L0P_CC_GC_3
AB15   | 225   AB15  D1.104   IO_L5P_FWE_B_2
AD11   | 226   AD11  D1.178   IO_L9P_CC_GC_4
P24   | 227   P24   D1.364   IO_L11N_CC_13
AA17   | 228   AA17  D1.100   IO_L3P_A21_2
R14   | 229   R14   D1.5   DXP_0
AB16   | 230   AB16  D1.105   IO_L5N_CSO_B_2
AC16   | 231   AC16  D1.165   IO_L2N_GC_D10_4
L20   | 232   L20   D1.228   IO_L11P_CC_SM14P_11
H13   | 233   H13   D1.64   IO_L1N_A16_1
D26   | 234   D26   D1.514   IO_L19P_15
AF2   | 235   AF2   D1.446   IO_L19P_14
AA20   | 236   AA20  D1.649   IO_L19P_17
G17   | 237   G17   D1.74   IO_L6N_A6_D22_1
AC26   | 238   AC26  D1.379   IO_L19P_13
P6   | 239   P6   D1.311   IO_L19P_12
N13   | 240   N13   D1.19   VREFN_0
F8   | 241   F8   D1.143   IO_L8P_GC_3
E17   | 242   E17   D1.138   IO_L5N_GC_3
N18   | 243   N18   D1.33   CS_B_0
AC7   | 244   AC7   D1.171   IO_L5N_GC_4
V6   | 245   V6   D1.676   IO_L6P_18
J19   | 246   J19   D1.205   IO_L6P_11
H4   | 247   H4   D1.271   IO_L6P_12
L2   | 248   L2   D1.406   IO_L6P_14
A18   | 249   A18   D1.475   IO_L6P_15
B11   | 250   B11   D1.541   IO_L6P_16
AA23   | 251   AA23  D1.610   IO_L6P_17
P5   | 252   P5   D1.305   IO_L16P_12
W25   | 253   W25   D1.373   IO_L16P_13
C2   | 254   C2   D1.575   IO_L16P_16
Y21   | 255   Y21   D1.643   IO_L16P_17
AB2   | 256   AB2   D1.440   IO_L16P_14
D24   | 257   D24   D1.508   IO_L16P_15
Y3   | 258   Y3   D1.675   IO_L5N_18
AF3   | 259   AF3   D1.710   IO_L16P_18
E15   | 260   E15   D1.134   IO_L3N_GC_3
Y13   | 261   Y13   D1.107   IO_L6N_D6_2
G16   | 262   G16   D1.69   IO_L4P_A11_D27_1
F20   | 263   F20   D1.194   IO_L0N_11
F7   | 264   F7   D1.260   IO_L0N_12
E1   | 265   E1   D1.395   IO_L0N_14
B14   | 266   B14   D1.464   IO_L0N_15
D10   | 267   D10   D1.530   IO_L0N_16
T22   | 268   T22   D1.599   IO_L0N_17
U4   | 269   U4   D1.665   IO_L0N_18
Y6   | 270   Y6   D1.680   IO_L8P_CC_18
K6   | 271   K6   D1.275   IO_L8P_CC_12
AC13   | 272   AC13  D1.176   IO_L8P_CC_GC_4
W10   | 273   W10   D1.60   TDO_0
D8   | 274   D8   D1.545   IO_L8P_CC_16
AC23   | 275   AC23  D1.614   IO_L8P_CC_17
M1   | 276   M1   D1.410   IO_L8P_CC_14
A20   | 277   A20   D1.479   IO_L8P_CC_15
H26   | 278   H26   D1.333   IO_L2N_SM6N_13
E20   | 279   E20   D1.196   IO_L1N_11
E5   | 280   E5   D1.262   IO_L1N_12
A15   | 281   A15   D1.466   IO_L1N_15
E3   | 282   E3   D1.397   IO_L1N_14
R20   | 283   R20   D1.601   IO_L1N_17
C12   | 284   C12   D1.532   IO_L1N_16
T4   | 285   T4   D1.667   IO_L1N_18
V11   | 286   V11   D1.58   TDI_0
N23   | 287   N23   D1.239   IO_L16N_SM12N_11
AA13   | 288   AA13  D1.112   IO_L9P_D1_FS1_2
N24   | 289   N24   D1.347   IO_L9N_CC_SM0N_13
A1   | 290   A1   A1.2   GND
AC11   | 291   AC11  D1.175   IO_L7N_GC_VRP_4
M20   | 292   M20   D1.236   IO_L15P_SM13P_11
E10   | 293   E10   D1.135   IO_L4P_GC_3
AD15   | 294   AD15  D1.168   IO_L4P_GC_4
AA4   | 295   AA4   D1.682   IO_L9P_CC_18
C19   | 296   C19   D1.481   IO_L9P_CC_15
M2   | 297   M2   D1.412   IO_L9P_CC_14
AB24   | 298   AB24  D1.616   IO_L9P_CC_17
B7   | 299   B7   D1.547   IO_L9P_CC_16
K21   | 300   K21   D1.211   IO_L9P_CC_11
N21   | 301   N21   D1.241   IO_L17N_SM11N_11
L7   | 302   L7   D1.277   IO_L9P_CC_12
Y12   | 303   Y12   D1.106   IO_L6P_D7_2
E18   | 304   E18   D1.141   IO_L7P_GC_3
E25   | 305   E25   D1.330   IO_L1P_SM7P_13
R22   | 306   R22   D1.242   IO_L18P_SM10P_11
M24   | 307   M24   D1.346   IO_L9P_CC_SM0P_13
H6   | 308   H6   D1.269   IO_L5P_12
H21   | 309   H21   D1.203   IO_L5P_11
V24   | 310   V24   D1.608   IO_L5P_17
B9   | 311   B9   D1.539   IO_L5P_16
B17   | 312   B17   D1.473   IO_L5P_15
H3   | 313   H3   D1.404   IO_L5P_14
W3   | 314   W3   D1.674   IO_L5P_18
AD10   | 315   AD10  D1.179   IO_L9N_CC_GC_4
K5   | 316   K5   D1.293   IO_L10P_CC_12
P26   | 317   P26   D1.361   IO_L10P_CC_13
P1   | 318   P1   D1.428   IO_L10P_CC_14
D21   | 319   D21   D1.496   IO_L10P_CC_15
D5   | 320   D5   D1.563   IO_L10P_CC_16
AB22   | 321   AB22  D1.631   IO_L10P_CC_17
Y7   | 322   Y7   D1.698   IO_L10P_CC_18
H15   | 323   H15   A1.1   VCCINT
C1   | 324   C1   D1.580   IO_L18N_16
AB19   | 325   AB19  D1.648   IO_L18N_17
AD1   | 326   AD1   D1.445   IO_L18N_14
C26   | 327   C26   D1.513   IO_L18N_15
R5   | 328   R5   D1.310   IO_L18N_12
AA25   | 329   AA25  D1.378   IO_L18N_13
F15   | 330   F15   D1.65   IO_L2P_A15_D31_1
AF4   | 331   AF4   D1.715   IO_L18N_18
T23   | 332   T23   D1.598   IO_L0P_17
L18   | 333   L18   D1.27   HSWAPEN_0
AB11   | 334   AB11  D1.111   IO_L8N_D2_FS2_2
E11   | 335   E11   D1.136   IO_L4N_GC_VREF_3
V23   | 336   V23   D1.609   IO_L5N_17
AD14   | 337   AD14  D1.169   IO_L4N_GC_VREF_4
G1   | 338   G1   D1.398   IO_L2P_14
B15   | 339   B15   D1.467   IO_L2P_15
C13   | 340   C13   D1.533   IO_L2P_16
T20   | 341   T20   D1.602   IO_L2P_17
E22   | 342   E22   D1.197   IO_L2P_11
G6   | 343   G6   D1.263   IO_L2P_12
T7   | 344   T7   D1.668   IO_L2P_18
M19   | 345   M19   D1.237   IO_L15N_SM13N_11
V22   | 346   V22   D1.636   IO_L12N_VRP_17
A5   | 347   A5   D1.568   IO_L12N_VRP_16
C22   | 348   C22   D1.501   IO_L12N_VRP_15
U1   | 349   U1   D1.433   IO_L12N_VRP_14
R26   | 350   R26   D1.366   IO_L12N_VRP_13
M6   | 351   M6   D1.298   IO_L12N_VRP_12
L22   | 352   L22   D1.231   IO_L12N_VRP_11
AC3   | 353   AC3   D1.703   IO_L12N_VRP_18
AB10   | 354   AB10  D1.162   IO_L1P_GC_D13_4
H9   | 355   H9   D1.79   IO_L9P_CC_A1_D17_1
AD5   | 356   AD5   D1.713   IO_L17N_18
A25   | 357   A25   D1.511   IO_L17N_15
AC1   | 358   AC1   D1.443   IO_L17N_14
AC19   | 359   AC19  D1.646   IO_L17N_17
A3   | 360   A3   D1.578   IO_L17N_16
Y26   | 361   Y26   D1.376   IO_L17N_13
T3   | 362   T3   D1.308   IO_L17N_12
C9   | 363   C9   D1.537   IO_L4P_16
Y8   | 364   Y8   D1.98   IO_L2P_A23_2
K3   | 365   K3   D1.402   IO_L4P_14
D18   | 366   D18   D1.471   IO_L4P_15
J6   | 367   J6   D1.267   IO_L4P_12
AA15   | 368   AA15  D1.108   IO_L7P_D5_2
G21   | 369   G21   D1.201   IO_L4P_11
AA9   | 370   AA9   D1.103   IO_L4N_VREF_FOE_B_MOSI_2
V4   | 371   V4   D1.672   IO_L4P_18
AB17   | 372   AB17  D1.101   IO_L3N_A20_2
F22   | 373   F22   D1.199   IO_L3P_11
J1   | 374   J1   D1.408   IO_L7P_14
Y23   | 375   Y23   D1.612   IO_L7P_17
A9   | 376   A9   D1.543   IO_L7P_16
AE3   | 377   AE3   D1.711   IO_L16N_18
F2   | 378   F2   D1.400   IO_L3P_14
U22   | 379   U22   D1.604   IO_L3P_17
A13   | 380   A13   D1.535   IO_L3P_16
AB1   | 381   AB1   D1.441   IO_L16N_14
U5   | 382   U5   D1.670   IO_L3P_18
C3   | 383   C3   D1.576   IO_L16N_16
Y20   | 384   Y20   D1.644   IO_L16N_17
W5   | 385   W5   D1.678   IO_L7P_18
P4   | 386   P4   D1.306   IO_L16N_12
W26   | 387   W26   D1.374   IO_L16N_13
L24   | 388   L24   D1.340   IO_L6P_SM3P_13
E12   | 389   E12   D1.131   IO_L2P_GC_VRN_3
F9   | 390   F9   D1.139   IO_L6P_GC_3
AD13   | 391   AD13  D1.172   IO_L6P_GC_4
D14   | 392   D14   D1.130   IO_L1N_CC_GC_3
G12   | 393   G12   D1.67   IO_L3P_A13_D29_1
H16   | 394   H16   D1.70   IO_L4N_VREF_A10_D26_1
AA5   | 395   AA5   D1.683   IO_L9N_CC_18
AC24   | 396   AC24  D1.617   IO_L9N_CC_17
A7   | 397   A7   D1.548   IO_L9N_CC_16
D19   | 398   D19   D1.482   IO_L9N_CC_15
N2   | 399   N2   D1.413   IO_L9N_CC_14
D13   | 400   D13   D1.129   IO_L1P_CC_GC_3
M7   | 401   M7   D1.278   IO_L9N_CC_12
K20   | 402   K20   D1.212   IO_L9N_CC_11
H12   | 403   H12   D1.68   IO_L3N_A12_D28_1
F13   | 404   F13   D1.62   IO_L0N_A18_1
AB14   | 405   AB14  D1.109   IO_L7N_D4_2
AA3   | 406   AA3   D1.701   IO_L11N_CC_18
T5   | 407   T5   D1.666   IO_L1P_18
R21   | 408   R21   D1.600   IO_L1P_17
C11   | 409   C11   D1.531   IO_L1P_16
AB21   | 410   AB21  D1.634   IO_L11N_CC_17
F3   | 411   F3   D1.396   IO_L1P_14
E6   | 412   E6   D1.261   IO_L1P_12
E21   | 413   E21   D1.195   IO_L1P_11
L3   | 414   L3   D1.296   IO_L11N_CC_12
AB4   | 415   AB4   D1.700   IO_L11P_CC_18
AC21   | 416   AC21  D1.633   IO_L11P_CC_17
C6   | 417   C6   D1.565   IO_L11P_CC_16
C21   | 418   C21   D1.498   IO_L11P_CC_15
T2   | 419   T2   D1.430   IO_L11P_CC_14
P25   | 420   P25   D1.363   IO_L11P_CC_13
L4   | 421   L4   D1.295   IO_L11P_CC_12
M26   | 422   M26   D1.345   IO_L8N_CC_SM1N_13
AA18   | 423   AA18  D1.96   IO_L1P_CC_A25_2
P18   | 424   P18   D1.34   RDWR_B_0
E7   | 425   E7   D1.259   IO_L0P_12
G20   | 426   G20   D1.193   IO_L0P_11
D11   | 427   D11   D1.529   IO_L0P_16
E26   | 428   E26   D1.331   IO_L1N_SM7N_13
E2   | 429   E2   D1.394   IO_L0P_14
C14   | 430   C14   D1.463   IO_L0P_15
A17   | 431   A17   D1.474   IO_L5N_15
J3   | 432   J3   D1.405   IO_L5N_14
V3   | 433   V3   D1.664   IO_L0P_18
B10   | 434   B10   D1.540   IO_L5N_16
H22   | 435   H22   D1.204   IO_L5N_11
G5   | 436   G5   D1.270   IO_L5N_12
J21   | 437   J21   D1.209   IO_L8P_CC_11
N4   | 438   N4   D1.304   IO_L15N_12
H11   | 439   H11   D1.71   IO_L5P_A9_D25_1
G10   | 440   G10   D1.75   IO_L7P_A5_D21_1
E16   | 441   E16   D1.137   IO_L5P_GC_3
AD8   | 442   AD8   D1.170   IO_L5P_GC_4
B5   | 443   B5   D1.569   IO_L13P_16
M14   | 444   M14   D1.11   AVDD_0
[Model Data]
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[End Model Data]
[End Package Model]
| End [Component] Virtex-5
| Models and submodels in the file (6): LVCMOS25_F_12_O (Output), LVCMOS25_S_12 (I/O), LVCMOS25_S_12_I (Input), LVDS_25 (I/O), LVDS_25_I (Input), LVDS_25_O (Output)
